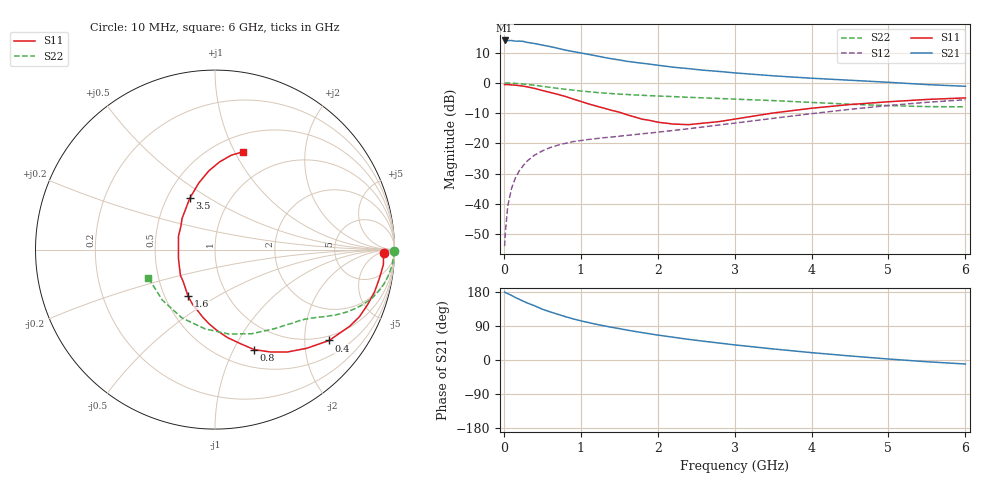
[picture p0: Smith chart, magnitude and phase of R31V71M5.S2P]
! SIEMENS Small Signal Semiconductors
! BFR181
! Si NPN RF Bipolar Junction Transistor in SOT23
! VCE = 1.75 V  IC = 1.5 mA
! Common Emitter S-Parameters:  May  1996
# GHz  S  MA  R  50
!  f  S11  S21  S12  S22
! GHz  MAG  ANG  MAG  ANG  MAG  ANG  MAG  ANG
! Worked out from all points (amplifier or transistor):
!   36 points, 10 MHz to 6 GHz, reference 50 ohm
!   highest |S21| = 14.1 dB at 10 MHz (marker M1)
!   |S21| within 3 dB of that: start of sweep to 770 MHz
!   unconditionally stable (mu >= 1): 1.714 GHz to 3.533 GHz
!   at 250 MHz: K = 0.20, MSG = 20.6 dB, |S12| = -27.4 dB
!   at 1.4 GHz: K = 0.89, MSG = 12.9 dB, |S12| = -17.9 dB
!   at 6 GHz: K = 0.87, MSG = 2.2 dB, |S12| = -5.5 dB
!   S11 on the Smith chart (normalised r, x): 10 MHz: 31, -9; 400 MHz: 0.87, -2.61; 800 MHz: 0.70, -1.21; 1.6 GHz: 0.66, -0.37; 3.5 GHz: 0.65, +0.41; 6 GHz: 0.67, +1.08
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0.01  0.9428 -1.0  5.046 179.4  0.002 93.4  0.9989 -0.5
0.02  0.9393 -2.1  4.961 177.9  0.0034 85.7  0.9953 -1.1
0.05  0.9419 -5.1  5.005 175.2  0.0091 87.3  0.995 -2.4
0.1  0.9295 -10.1  5.039 170.5  0.0181 82.6  0.9917 -4.7
0.15  0.9193 -14.9  4.909 164.9  0.0268 80.3  0.9823 -7.1
0.25  0.887 -25.0  4.876 155.4  0.0427 74.0  0.9608 -11.5
0.3  0.8638 -29.6  4.692 150.9  0.0508 72.1  0.947 -13.5
0.4  0.8131 -38.5  4.487 143.0  0.0642 67.2  0.9177 -17.0
0.5  0.7507 -47.1  4.234 134.1  0.0753 63.2  0.8815 -20.2
0.6  0.699 -54.7  4.005 127.2  0.0853 59.4  0.8463 -22.9
0.8  0.5984 -68.6  3.499 114.4  0.1005 53.9  0.7865 -27.0
0.9  0.5436 -74.8  3.306 108.6  0.1071 52.3  0.762 -28.6
1.1  0.4512 -88.5  2.973 98.8  0.1162 50.1  0.7165 -31.4
1.3  0.3835 -100.1  2.652 90.3  0.1244 48.8  0.6814 -33.6
1.6  0.2982 -120.4  2.281 78.9  0.1357 48.6  0.6448 -36.7
1.9  0.2402 -143.2  2.045 69.0  0.1485 49.9  0.6155 -40.0
2.2  0.2093 -166.8  1.824 60.2  0.1637 50.9  0.5952 -43.6
2.8  0.2298 145.9  1.55 44.7  0.2022 52.8  0.5542 -52.3
3.5  0.3186 116.2  1.313 29.2  0.2599 51.8  0.5109 -66.6
4.5  0.4399 94.5  1.109 10.7  0.3666 44.7  0.4451 -97.2
5.5  0.5337 80.2  0.94 -4.6  0.4787 32.2  0.4065 -136.5
6  0.5666 74.1  0.881 -10.6  0.5284 24.5  0.4033 -157.2
